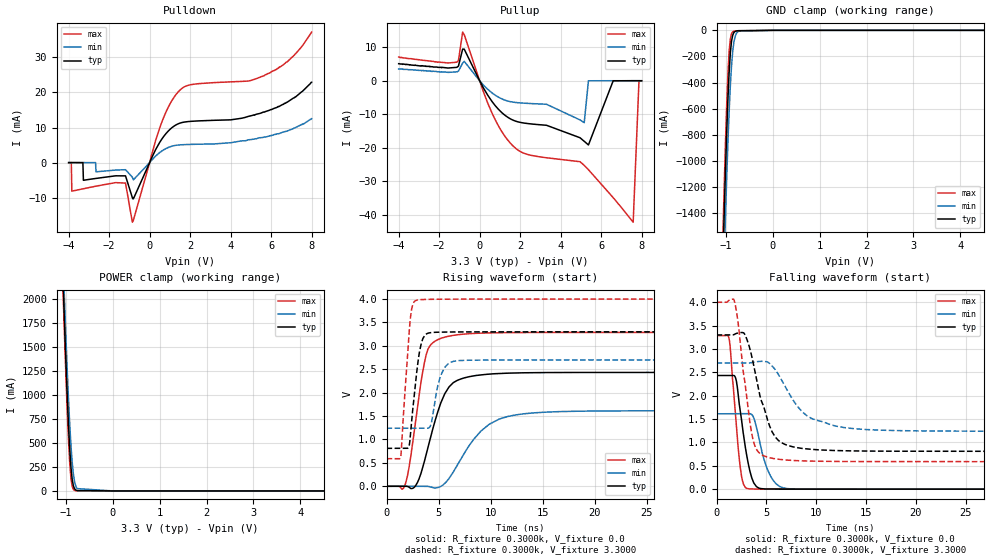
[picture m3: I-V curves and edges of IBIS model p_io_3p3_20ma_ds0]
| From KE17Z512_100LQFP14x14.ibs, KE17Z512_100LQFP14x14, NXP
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[Model] p_io_3p3_20ma_ds0
|   Model p_io_3p3_20ma_ds0
| This model was characterised for following simulation conditions:
| External (pad) voltage:
|   - Typ: 3.3V,   - Min: 2.7V,   - Max: 4.0V
| Library cells for typ/min/max conditions are connected as defined below:
|  pad - External Pad
|  ipp_do_lv - Core Input
|  ipp_obe_lv - Output Buffer Enable
|  abt_close_nor_rst_mv - vdde
|  dvdd - dvdd
|  dvss - dvss
|  esd_boost - vdde
|  ipp_dse_lv - dvss
|  ipp_ina_280_mv - NC
|  ipp_ina_40_a_mv - NC
|  ipp_ina_40_b_mv - NC
|  ipp_ina_40_c_mv - NC
|  ipp_ina_40_d_mv - NC
|  ipp_ina_40_e_mv - NC
|  ipp_ina_40_f_mv - NC
|  ipp_ina_40_g_mv - NC
|  ipp_ina_40_h_mv - NC
|  ipp_ind_lv - NC
|  vdde - vdde
|  vsse - vsse
| All other pins connected to ground
Model_type I/O
Polarity   Non-Inverting
Enable   Active-High
Vinl =   0.9900V
Vinh =   2.3100V
Vmeas =  1.6500V
Cref =   50.0000F
C_comp   2.8325pF   2.6979pF   3.0285pF
[Model Spec]
| variable   typ   min   max
Vinh   2.3100V   1.8900V   2.8000V
Vinl   0.9900V   0.8100V   1.2000V
S_overshoot_high   3.6000V   3.0000V   4.3000V
S_overshoot_low   -0.3000V   -0.3000V   -0.3000V
Vmeas   1.6500V   1.3500V   2.0000V
[Temperature Range]   25.0000   0.1250k   -40.0000
[Voltage Range]   3.3000V   2.7000V   4.0000V
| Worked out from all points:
|   slope of the pulldown table from 0 to 0.495 V, typ, clamps not added: 86.1 ohm
|   slope of the pullup table from 0 to 0.495 V, typ, clamps not added: 95.9 ohm
|   rising waveform, R_fixture 0.3000k, V_fixture 0.0: 20-80 % time 1.95ns typ, 3.22ns min, 1.29ns max; typ from 0 V to 2.43 V
|   rising waveform, R_fixture 0.3000k, V_fixture 3.3000: 20-80 % time 737ps typ, 841ps min, 627ps max; typ from 0.81 V to 3.3 V
|   falling waveform, R_fixture 0.3000k, V_fixture 0.0: 20-80 % time 1.03ns typ, 1.28ns min, 774ps max; typ from 2.43 V to 0 V
|   falling waveform, R_fixture 0.3000k, V_fixture 3.3000: 20-80 % time 1.83ns typ, 3.04ns min, 1.16ns max; typ from 3.3 V to 0.81 V
[Pulldown]
|Voltage   I(typ)   I(min)   I(max)
-4V       10uA       10uA       -80uA
-3.87V    10uA       10uA       -90uA
-3.844V   0A         10uA       -8.14mA
-3.298V   -10uA      0A         -7.48mA
-3.272V   -5.04mA    10uA       -7.45mA
-1.192V   -3.779mA   -2.025mA   -5.84mA
-854mV    -10mA      -4.159mA   -16.99mA
498mV     5.783mA    2.872mA    9.907mA
1.434V    11.11mA    5.018mA    20.3mA
5.672V    14.4mA     7.3mA      24.8mA
6.79V     17.2mA     9mA        28.7mA
8V        22.9mA     12.5mA     37.2mA
[Pullup]
|Voltage   I(typ)   I(min)   I(max)
-4V       5.1mA      3.5mA      7.1mA
-1.126V   4.01mA     2.66mA     5.55mA
-840mV    9.451mA    5.276mA    14.53mA
616mV     -6.231mA   -3.647mA   -9.711mA
1.526V    -11.39mA   -6.242mA   -18.68mA
3.3V      -13.28mA   -7.01mA    -22.99mA
5.166V    -18.07mA   -12.5mA    -25.25mA
5.374V    -19.16mA   0A         -26.55mA
6.596V    -10uA      10uA       -34.89mA
7.584V    20uA       10uA       -42.22mA
7.87V     20uA       10uA       -90uA
8V        20uA       0A         -80uA
[GND_clamp]
|Voltage   I(typ)   I(min)   I(max)
-4V       -49.59A    -49.54A    -49.68A
-1.062V   -1.74A     -2.082A    -1.538A
-1.036V   -1.402A    -1.75A     -1.192A
-1.01V    -1.083A    -1.435A    -869.2mA
-984mV    -791.3mA   -1.14A     -579.3mA
-958mV    -535mA     -869mA     -338.2mA
-932mV    -326.2mA   -629.6mA   -164.5mA
-906mV    -175.2mA   -428.2mA   -66.24mA
-880mV    -83.05mA   -270.6mA   -25.06mA
-828mV    -16.12mA   -86.77mA   -7.14mA
-724mV    -2.673mA   -6.605mA   -3.909mA
8V        0A         0A         0A
[POWER_clamp]
|Voltage   I(typ)   I(min)   I(max)
-4V       52.67A     52.45A     52.88A
-1.074V   2.381A     2.6A       2.272A
-1.048V   2.004A     2.236A     1.882A
-1.022V   1.639A     1.885A     1.505A
-970mV    970.2mA    1.235A     814mA
-918mV    434.5mA    688.7mA    285.8mA
-892mV    245.5mA    470.7mA    127mA
-866mV    120.4mA    298.4mA    45.78mA
-814mV    21.03mA    94.6mA     5.402mA
-762mV    3.719mA    24.12mA    1.768mA
0V        97.57pA    2.637nA    84.84pA
8V        0A         0A         0A
[Ramp]
| variable   typ   min   max
dV/dt_r  1.4597/1.9485n   0.9680/3.2184n   1.9722/1.2863n
dV/dt_f  1.4937/1.8347n   0.8757/3.0424n   2.0462/1.1640n
R_load = 0.3000k
[Rising Waveform]
R_fixture= 0.3000k
V_fixture= 0.0
V_fixture_min= 0.0
V_fixture_max= 0.0
|time   V(typ)   V(min)   V(max)
0s        178.7pV    57.84nV    702.6pV
1.772ns   270.5uV    7.879uV    25.56mV
2.267ns   -37.08mV   38.7uV     544.7mV
2.8ns     15.36mV    60.05uV    1.413V
3.8ns     671mV      305uV      2.804V
5.289ns   1.823V     8.293mV    3.166V
6.762ns   2.259V     440.3mV    3.236V
9.056ns   2.38V      1.178V     3.272V
11.65ns   2.417V     1.492V     3.283V
40ns      2.433V     1.613V     3.287V
[Rising Waveform]
R_fixture= 0.3000k
V_fixture= 3.3000
V_fixture_min= 2.7000
V_fixture_max= 4.0000
|time   V(typ)   V(min)   V(max)
0s        810.5mV    1.24V      589.7mV
1.359ns   811mV      1.241V     631.1mV
2.243ns   972.4mV    1.241V     3.49V
2.849ns   2.336V     1.241V     3.974V
3.173ns   2.885V     1.241V     3.986V
3.673ns   3.226V     1.241V     3.992V
4.259ns   3.283V     1.315V     3.995V
5.42ns    3.294V     2.472V     3.998V
6.6ns     3.297V     2.676V     3.999V
40ns      3.3V       2.7V       4V
[Falling Waveform]
R_fixture= 0.3000k
V_fixture= 0.0
V_fixture_min= 0.0
V_fixture_max= 0.0
|time   V(typ)   V(min)   V(max)
0s        2.433V     1.613V     3.287V
1.269ns   2.433V     1.613V     3.21V
1.936ns   2.364V     1.613V     1.47V
2.336ns   1.743V     1.613V     539.3mV
2.577ns   1.365V     1.613V     198.1mV
3.013ns   741.9mV    1.614V     19.2mV
3.986ns   57.14mV    1.339V     2.778mV
5.229ns   3.199mV    363.1mV    1.159mV
6.69ns    1.209mV    27.32mV    489.7uV
40ns      216.1nV    659.8nV    94.46nV
[Falling Waveform]
R_fixture= 0.3000k
V_fixture= 3.3000
V_fixture_min= 2.7000
V_fixture_max= 4.0000
|time   V(typ)   V(min)   V(max)
0s        3.3V       2.7V       4V
1.797ns   3.313V     2.7V       4.022V
2.777ns   3.333V     2.7V       2.385V
3.623ns   2.756V     2.714V     1.09V
4.93ns    1.617V     2.73V      698.5mV
5.881ns   1.118V     2.562V     650.4mV
6.789ns   964.5mV    2.235V     626.9mV
9.121ns   859.6mV    1.562V     602.4mV
12.21ns   824.9mV    1.339V     593mV
40ns      810.5mV    1.24V      589.7mV
